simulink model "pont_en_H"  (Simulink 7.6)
settings: Solver=ode15s  StartTime=0.0  StopTime=N  FixedStep=0.0001  RelTol=1e-3
InitFcn:
  | clear all, clc
  | N=0.1;
StopFcn:
  | close all, clc
  | load Pont_en_H.mat
  | [AX,H1,H2] = plotyy(x(1,:),x(2,:),x(1,:),x(3,:),'plot');
  | set(get(AX(1),'Ylabel'),'String','Vitesse angulaire')
  | set(get(AX(2),'Ylabel'),'String','Position angulaire')
  | xlabel('temps')
  | title('Position et vitesse angulaires - Moteur CC, Pont en H')
  | grid
  | %axis([0 N -0.2 1.2])
  | delete *.mat
undefined symbols (not defined in the file or in its folder): sigbuilder_block
libraries: elec_lib x15, fl_lib x15, nesl_utility x6

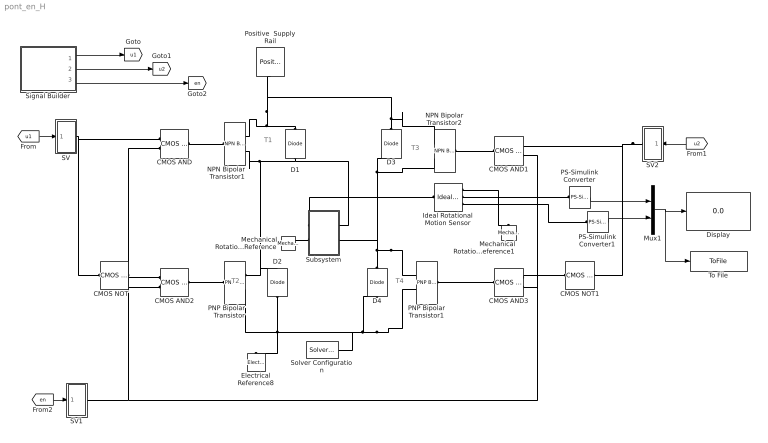
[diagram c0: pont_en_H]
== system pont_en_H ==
  note: T1
  note: T2
  note: T3
  note: T4
  CMOS AND{,1..3} (4 alike) : elec_lib/Integrated Circuits/Logic/CMOS AND  DialogController=NetworkEngine.DynNeDlgSource  SystemSampleTime=-1  V_IL=2 V  V_IH=3 V  C_IN=5 pF  output_type=1  V_OL=0 V  V_OH=5 V  V_CC=5 V  V_meas=5 V  R_OUT=25 Ohm  R_OH=[ 25 250 ] Ohm  I_OH=63 mA  R_OL=[ 30 800 ] Ohm  I_OL=-45 mA  Delay=25 ns  Ron=5 Ohm  Vf=0.6 V  output_state=1  LocalVarLogging=[]
  CMOS NOT : elec_lib/Integrated Circuits/Logic/CMOS NOT  DialogController=NetworkEngine.DynNeDlgSource  SystemSampleTime=-1  V_IL=2 V  V_IH=3 V  C_IN=5 pF  output_type=1  V_OL=0 V  V_OH=5 V  V_CC=5 V  V_meas=5 V  R_OUT=25 Ohm  R_OH=[ 25 250 ] Ohm  I_OH=63 mA  R_OL=[ 30 800 ] Ohm  I_OL=-45 mA  Delay=25 ns  Ron=5 Ohm  Vf=0.6 V  output_state=1  LocalVarLogging=[]
  CMOS NOT1 : elec_lib/Integrated Circuits/Logic/CMOS NOT  DialogController=NetworkEngine.DynNeDlgSource  SystemSampleTime=-1  V_IL=2 V  V_IH=3 V  C_IN=5 pF  output_type=1  V_OL=0 V  V_OH=5 V  V_CC=5 V  V_meas=5 V  R_OUT=25 Ohm  R_OH=[ 25 250 ] Ohm  I_OH=63 mA  R_OL=[ 30 800 ] Ohm  I_OL=-45 mA  Delay=25 ns  Ron=5 Ohm  Vf=0.6 V  output_state=1  LocalVarLogging=[]
  D{1..4} (4 alike) : elec_lib/Semiconductor Devices/Diode  DialogController=NetworkEngine.DynNeDlgSource  SystemSampleTime=-1  ModelType=1  Vf=0.6 V  Ron=0.3 Ohm  Goff=1e-8 S  Rz=0.3 Ohm  Vz=50 V  C_PWL=5 pF  prmExp=1  I12=[ 0.07 1.5 ] A  V12=[ 0.7 0.8 ] V  I1=0.07 A  V1=0.7 V  RS=0.01 Ohm  IS=1e-14 A  Tmeas=25 C  ec=1  BV=Inf V  C_param=1  CJ0=5 pF  VJ=1 V  Mgrad=0.5  Vvec=[ 0.1 10 100 ] V  Cvec=[ 3.5 1 0.4 ] pF  FC=0.5  LocalVarLogging=[]
  Display : Display
  Electrical Reference8 : fl_lib/Electrical/Electrical Elements/Electrical Reference  DialogController=NetworkEngine.DynNeDlgSource  SystemSampleTime=-1  i_Log=off  LocalVarNames=|i  LocalVarDescs=|i  LocalVarLogging=[]
  Ideal Rotational Motion Sensor : fl_lib/Mechanical/Mechanical Sensors/Ideal Rotational Motion Sensor  DialogController=NetworkEngine.DynNeDlgSource  SystemSampleTime=-1  offset=0 rad  w_Log=off  t_Log=off  phi_Log=off  LocalVarNames=|w|t|phi  LocalVarDescs=|w|t|phi  LocalVarLogging=[0 0 0]
  Mechanical Rotational Reference : fl_lib/Mechanical/Rotational Elements/Mechanical Rotational Reference  DialogController=NetworkEngine.DynNeDlgSource  SystemSampleTime=-1  t_Log=off  LocalVarNames=|t  LocalVarDescs=|t  LocalVarLogging=0
  Mechanical Rotational Reference1 : fl_lib/Mechanical/Rotational Elements/Mechanical Rotational Reference  DialogController=NetworkEngine.DynNeDlgSource  SystemSampleTime=-1  t_Log=off  LocalVarNames=|t  LocalVarDescs=|t  LocalVarLogging=0
  Mux1 : Mux  Inputs=2
  NPN Bipolar Transistor1 : elec_lib/Semiconductor Devices/NPN Bipolar Transistor  DialogController=NetworkEngine.DynNeDlgSource  SystemSampleTime=-1  parameterization=1  BF=100  IS=1e-14 A  VAF=200 V  hfe=100  hoe=5e-5 1/Ohm  Ic_h=1 mA  V1=0.55 V  I1=0.5 mA  BR=1  Tmeas=25 C  RC=0.01 Ohm  RE=1e-4 Ohm  RB=1 Ohm  C_BC=5 pF  C_BE=5 pF  TF=0 us  TR=0 us  LocalVarLogging=[]
  NPN Bipolar Transistor2 : elec_lib/Semiconductor Devices/NPN Bipolar Transistor  DialogController=NetworkEngine.DynNeDlgSource  SystemSampleTime=-1  parameterization=1  BF=100  IS=1e-14 A  VAF=200 V  hfe=100  hoe=5e-5 1/Ohm  Ic_h=1 mA  V1=0.55 V  I1=0.5 mA  BR=1  Tmeas=25 C  RC=0.01 Ohm  RE=1e-4 Ohm  RB=1 Ohm  C_BC=5 pF  C_BE=5 pF  TF=0 us  TR=0 us  LocalVarLogging=[]
  PNP Bipolar Transistor : elec_lib/Semiconductor Devices/PNP Bipolar Transistor  DialogController=NetworkEngine.DynNeDlgSource  SystemSampleTime=-1  parameterization=1  BF=100  IS=1e-14 A  VAF=200 V  hfe=100  hoe=5e-5 1/Ohm  Ic_h=1 mA  V1=0.55 V  I1=0.5 mA  BR=1  Tmeas=25 C  RC=0.01 Ohm  RE=1e-4 Ohm  RB=1 Ohm  C_BC=5 pF  C_BE=5 pF  TF=0 us  TR=0 us  LocalVarLogging=[]
  PNP Bipolar Transistor1 : elec_lib/Semiconductor Devices/PNP Bipolar Transistor  DialogController=NetworkEngine.DynNeDlgSource  SystemSampleTime=-1  parameterization=1  BF=100  IS=1e-14 A  VAF=200 V  hfe=100  hoe=5e-5 1/Ohm  Ic_h=1 mA  V1=0.55 V  I1=0.5 mA  BR=1  Tmeas=25 C  RC=0.01 Ohm  RE=1e-4 Ohm  RB=1 Ohm  C_BC=5 pF  C_BE=5 pF  TF=0 us  TR=0 us  LocalVarLogging=[]
  PS-Simulink Converter : nesl_utility/PS-Simulink Converter  DialogController=NetworkEngine.DynNeUtilDlgSource  SystemSampleTime=-1  PhysicalDomain=network_engine_domain  LeftPortType=input  RightPortType=output  SubClassName=ps_output  Unit=1  AffineConversion=off
  PS-Simulink Converter1 : nesl_utility/PS-Simulink Converter  DialogController=NetworkEngine.DynNeUtilDlgSource  SystemSampleTime=-1  PhysicalDomain=network_engine_domain  LeftPortType=input  RightPortType=output  SubClassName=ps_output  Unit=1  AffineConversion=off
  Positive  Supply Rail : elec_lib/Sources/Positive Supply Rail  DialogController=NetworkEngine.DynNeDlgSource  SystemSampleTime=-1  v0=50 V  current_Log=off  voltage_Log=off  power_Log=off  LocalVarNames=|current|voltage|power  LocalVarDescs=|Current (A)|Voltage (V)|Power (W)  LocalVarLogging=[0 0 0]
  SV : Subsystem
  SV1 : Subsystem
  SV2 : Subsystem
  Signal Builder : Subsystem  Tag=STV Subsys  LoadFcn=sigbuilder_block('load');  StartFcn=sigbuilder_block('start');  StopFcn=sigbuilder_block('stop');  ClipboardFcn=sigbuilder_block('clipboard');
  Solver Configuration : nesl_utility/Solver Configuration  DialogController=NetworkEngine.DynNeUtilDlgSource  SystemSampleTime=-1  PhysicalDomain=network_engine_domain  LeftPortType=input  RightPortType=generic  SubClassName=solver  Accelerate=off  Profile=off  ResidualTolerance=1e-9  MaxNonlinIter=3  MaxModeIter=2  DoFixedCost=off  UseLocalSampling=off  DoDC=off  LinearAlgebra=Sparse  LocalSolverSampleTime=.001  LocalSolverChoice=NE_BACKWARD_EULER_ADVANCER  UseLocalSolver=off
  Subsystem : Subsystem
  To File : ToFile  Filename=Pont_en_H  MatrixName=x
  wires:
  [en] -> SV1/1(S)
  [u2] -> SV2/1(S)
  PS-Simulink Converter/1 -> Mux1/1
  Mux1/1 -> Display/1, To File/1
  PS-Simulink Converter1/1 -> Mux1/2
  [u1] -> SV/1(S)
  Signal Builder/1(Signal 5) -> [u1]
  Signal Builder/2(Signal 6) -> [u2]
  Signal Builder/3(Signal 1) -> [en]
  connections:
  D1/LConn1 -- NPN Bipolar Transistor1/RConn2 -- PNP Bipolar Transistor/RConn1 -- D2/RConn1 -- Subsystem/LConn1
  D3/RConn1 -- Positive  Supply Rail/RConn1 -- NPN Bipolar Transistor1/RConn1 -- D1/RConn1 -- NPN Bipolar Transistor2/RConn1
  PNP Bipolar Transistor1/RConn1 -- D3/LConn1 -- NPN Bipolar Transistor2/RConn2 -- D4/RConn1 -- Subsystem/LConn2
  PNP Bipolar Transistor1/RConn2 -- D4/LConn1 -- D2/LConn1 -- PNP Bipolar Transistor/RConn2 -- Electrical Reference8/LConn1 -- Solver Configuration/RConn1
  NPN Bipolar Transistor1/LConn1 -- CMOS AND/RConn1
  CMOS AND1/RConn1 -- NPN Bipolar Transistor2/LConn1
  SV/RConn1 -- CMOS AND/LConn1 -- CMOS NOT/LConn1
  CMOS NOT/RConn1 -- CMOS AND2/LConn1
  CMOS AND2/RConn1 -- PNP Bipolar Transistor/LConn1
  PNP Bipolar Transistor1/LConn1 -- CMOS AND3/RConn1
  CMOS AND3/LConn1 -- CMOS NOT1/RConn1
  SV2/RConn1 -- CMOS AND1/LConn1 -- CMOS NOT1/LConn1
  SV1/RConn1 -- CMOS AND1/LConn2 -- CMOS AND3/LConn2 -- CMOS AND/LConn2 -- CMOS AND2/LConn2
  Ideal Rotational Motion Sensor/LConn1 -- Subsystem/RConn1
  Ideal Rotational Motion Sensor/RConn1 -- Mechanical Rotational Reference1/LConn1
  Ideal Rotational Motion Sensor/RConn2 -- PS-Simulink Converter/LConn1
  Ideal Rotational Motion Sensor/RConn3 -- PS-Simulink Converter1/LConn1
  Mechanical Rotational Reference/LConn1 -- Subsystem/RConn2

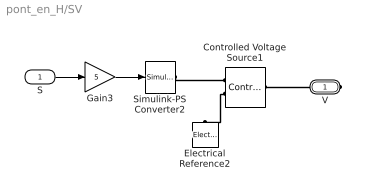
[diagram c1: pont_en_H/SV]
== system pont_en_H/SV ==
  S : Inport
  Controlled Voltage Source1 : fl_lib/Electrical/Electrical Sources/Controlled Voltage Source  DialogController=NetworkEngine.DynNeDlgSource  SystemSampleTime=-1  i_Log=off  v_Log=off  LocalVarNames=|i|v  LocalVarDescs=|i|v  LocalVarLogging=[0 0]
  Electrical Reference2 : fl_lib/Electrical/Electrical Elements/Electrical Reference  DialogController=NetworkEngine.DynNeDlgSource  SystemSampleTime=-1  i_Log=off  LocalVarNames=|i  LocalVarDescs=|i  LocalVarLogging=[]
  Gain3 : Gain  Gain=5
  Simulink-PS Converter2 : nesl_utility/Simulink-PS Converter  DialogController=NetworkEngine.DynNeUtilDlgSource  SystemSampleTime=-1  PhysicalDomain=network_engine_domain  LeftPortType=input  RightPortType=output  SubClassName=ps_input  Unit=1  AffineConversion=off  InputFilterTimeConstant=.001  UdotUserProvided=0
  V : PMIOPort  Port=1  Side=Right
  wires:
  S/1 -> Gain3/1
  Gain3/1 -> Simulink-PS Converter2/1
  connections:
  V/RConn1 -- Controlled Voltage Source1/LConn1
  Controlled Voltage Source1/RConn2 -- Electrical Reference2/LConn1
  Simulink-PS Converter2/RConn1 -- Controlled Voltage Source1/RConn1

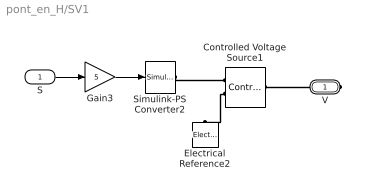
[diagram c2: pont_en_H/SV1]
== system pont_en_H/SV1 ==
  S : Inport
  Controlled Voltage Source1 : fl_lib/Electrical/Electrical Sources/Controlled Voltage Source  DialogController=NetworkEngine.DynNeDlgSource  SystemSampleTime=-1  i_Log=off  v_Log=off  LocalVarNames=|i|v  LocalVarDescs=|i|v  LocalVarLogging=[0 0]
  Electrical Reference2 : fl_lib/Electrical/Electrical Elements/Electrical Reference  DialogController=NetworkEngine.DynNeDlgSource  SystemSampleTime=-1  i_Log=off  LocalVarNames=|i  LocalVarDescs=|i  LocalVarLogging=[]
  Gain3 : Gain  Gain=5
  Simulink-PS Converter2 : nesl_utility/Simulink-PS Converter  DialogController=NetworkEngine.DynNeUtilDlgSource  SystemSampleTime=-1  PhysicalDomain=network_engine_domain  LeftPortType=input  RightPortType=output  SubClassName=ps_input  Unit=1  AffineConversion=off  InputFilterTimeConstant=.001  UdotUserProvided=0
  V : PMIOPort  Port=1  Side=Right
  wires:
  Gain3/1 -> Simulink-PS Converter2/1
  S/1 -> Gain3/1
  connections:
  Simulink-PS Converter2/RConn1 -- Controlled Voltage Source1/RConn1
  Controlled Voltage Source1/RConn2 -- Electrical Reference2/LConn1
  V/RConn1 -- Controlled Voltage Source1/LConn1

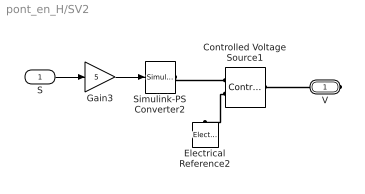
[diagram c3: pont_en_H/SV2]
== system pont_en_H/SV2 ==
  S : Inport
  Controlled Voltage Source1 : fl_lib/Electrical/Electrical Sources/Controlled Voltage Source  DialogController=NetworkEngine.DynNeDlgSource  SystemSampleTime=-1  i_Log=off  v_Log=off  LocalVarNames=|i|v  LocalVarDescs=|i|v  LocalVarLogging=[0 0]
  Electrical Reference2 : fl_lib/Electrical/Electrical Elements/Electrical Reference  DialogController=NetworkEngine.DynNeDlgSource  SystemSampleTime=-1  i_Log=off  LocalVarNames=|i  LocalVarDescs=|i  LocalVarLogging=[]
  Gain3 : Gain  Gain=5
  Simulink-PS Converter2 : nesl_utility/Simulink-PS Converter  DialogController=NetworkEngine.DynNeUtilDlgSource  SystemSampleTime=-1  PhysicalDomain=network_engine_domain  LeftPortType=input  RightPortType=output  SubClassName=ps_input  Unit=1  AffineConversion=off  InputFilterTimeConstant=.001  UdotUserProvided=0
  V : PMIOPort  Port=1  Side=Right
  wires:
  S/1 -> Gain3/1
  Gain3/1 -> Simulink-PS Converter2/1
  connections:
  V/RConn1 -- Controlled Voltage Source1/LConn1
  Controlled Voltage Source1/RConn2 -- Electrical Reference2/LConn1
  Simulink-PS Converter2/RConn1 -- Controlled Voltage Source1/RConn1

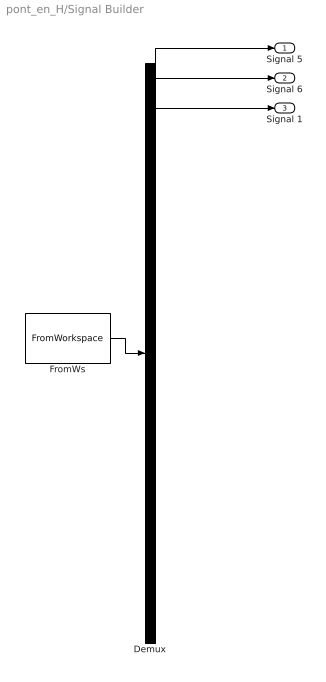
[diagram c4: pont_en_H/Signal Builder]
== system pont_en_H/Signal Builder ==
  Demux : Demux  Tag=STV Demux  Outputs=3
  FromWs : FromWorkspace  Tag=STV FromWs  VariableName=tuvar  SampleTime=0  SigBuilderData=DataTag0  VnvData=DataTag1
  Signal 5 : Outport  Tag=STV Outport
  Signal 6 : Outport  Tag=STV Outport  Port=2
  Signal 1 : Outport  Tag=STV Outport  Port=3
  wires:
  FromWs/1 -> Demux/1
  Demux/1 -> Signal 5/1
  Demux/2 -> Signal 6/1
  Demux/3 -> Signal 1/1

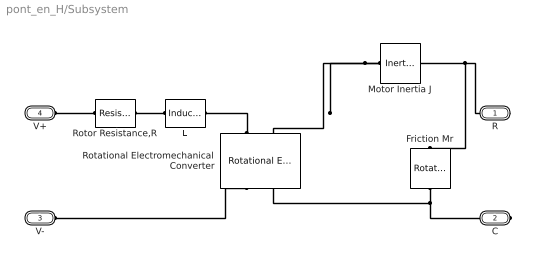
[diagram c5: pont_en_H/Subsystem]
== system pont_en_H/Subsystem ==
  Friction Mr : fl_lib/Mechanical/Rotational Elements/Rotational Friction  DialogController=NetworkEngine.DynNeDlgSource  SystemSampleTime=-1  brkwy_trq=0.01e-6 N*m  Col_trq=0.02e-12 N*m  visc_coef=0 N*m/(rad/s)  trans_coef=10 s/rad  vel_thr=0.1 rad/s  t_Log=off  w_Log=off  LocalVarNames=|friction_torque|rel_velocity|power  LocalVarDescs=|Friction torque (N*m)|Relative velocity (rad/s)|Power (W)  LocalVarLogging=[0 0 0]
  L : fl_lib/Electrical/Electrical Elements/Inductor  DialogController=NetworkEngine.DynNeDlgSource  SystemSampleTime=-1  l=12e-6 H  i0=0 A  r=0 Ohm  g=1e-09 1/Ohm  i_Log=off  v_Log=off  i_L_Log=off  LocalVarNames=|current|voltage|power  LocalVarDescs=|Inductor current (A) |Voltage across inductor (V)|Power (W)  LocalVarLogging=[0 0 0]
  Motor Inertia J : fl_lib/Mechanical/Rotational Elements/Inertia  DialogController=NetworkEngine.DynNeDlgSource  SystemSampleTime=-1  inertia=0.001 g*cm^2  initial_velocity=0 rad/s  t_Log=off  LocalVarNames=|torque|velocity  LocalVarDescs=|Inertia torque (N*m)|Inertia absolute velocity (rad/s)  LocalVarLogging=[0 0]
  Rotational Electromechanical Converter : fl_lib/Electrical/Electrical Elements/Rotational Electromechanical Converter  DialogController=NetworkEngine.DynNeDlgSource  SystemSampleTime=-1  K=0.072e-3*60/(2*pi) s*V/rad  i_Log=off  v_Log=off  t_Log=off  w_Log=off  LocalVarNames=|current|voltage|power|torque|speed  LocalVarDescs=|Current (A)|Voltage (V)|Power (W)|Torque (Nm)|Angular speed (rad/s)  LocalVarLogging=[0 0 0 0 0]
  Rotor Resistance,R : fl_lib/Electrical/Electrical Elements/Resistor  Tag=Factory Generic  DialogController=NetworkEngine.DynNeDlgSource  SystemSampleTime=-1  R=3.9 Ohm  i_Log=off  v_Log=off  LocalVarNames=|current|voltage|power  LocalVarDescs=|Resistor current (A)|Voltage across resistor (V)|Power (W)  LocalVarLogging=[0 0 0]
  R : PMIOPort  Port=1  Side=Right
  C : PMIOPort  Port=2  Side=Right
  V- : PMIOPort  Port=3  Side=Left
  V+ : PMIOPort  Port=4  Side=Left
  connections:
  Motor Inertia J/LConn1 -- Friction Mr/LConn1 -- R/RConn1 -- Rotational Electromechanical Converter/LConn2
  Friction Mr/RConn1 -- C/RConn1 -- Rotational Electromechanical Converter/RConn2
  L/LConn1 -- Rotor Resistance,R/RConn1
  Rotational Electromechanical Converter/LConn1 -- L/RConn1
  V-/RConn1 -- Rotational Electromechanical Converter/RConn1
  Rotor Resistance,R/LConn1 -- V+/RConn1
